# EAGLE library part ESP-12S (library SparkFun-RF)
AI-Thinker ESP-12S ESP-12S WiFi module is developed by AI-Thinker Co.,Ltd, core processor ESP8266 in smaller sizes of the module encapsulates Tensilica L106 integrates industry-leading ultra low power 32-bit MCU micro, with the 16-bit short mode, clock speed support 80 MHz, 160 MHz, supports the RTOS, integrated Wi-Fi MAC/BB/RF/PA/LNA, on-board antennas.
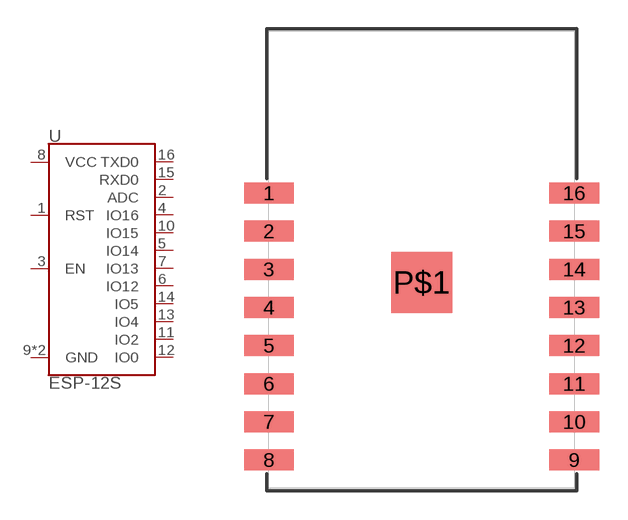
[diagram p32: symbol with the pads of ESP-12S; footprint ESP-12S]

Designator prefix U

## ESP-12S (PROD_ID: IC-14115)  [ESP-12S]
1  RST
2  ADC
3  EN
4  IO16
5  IO14
6  IO12
7  IO13
8  VCC
9  GND
10  IO15
11  IO2
12  IO0
13  IO4
14  IO5
15  RXD0
16  TXD0
P$1  GND

## Footprint ESP-12S (pad centres in mm)
smd 2.6 x 1.1: 1 -8,3.5; 2 -8,1.5; 3 -8,-0.5; 4 -8,-2.5; 5 -8,-4.5; 6 -8,-6.5; 7 -8,-8.5; 8 -8,-10.5; 9 8,-10.5; 10 8,-8.5; 11 8,-6.5; 12 8,-4.5; 13 8,-2.5; 14 8,-0.5; 15 8,1.5; 16 8,3.5
smd 3.2 x 3.2: P$1 0,-1.2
